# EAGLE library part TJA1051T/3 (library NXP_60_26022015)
High-speed CAN transceiver The TJA1051 is a high-speed CAN transceiver that provides an interface between a Controller Area Network (CAN) protocol controller and the physical two-wire CAN bus. The transceiver is designed for high-speed (up to 1 Mbit/s) CAN applications in the automotive industry, providing differential transmit and receive capability to (a microcontroller with) a CAN protocol controller. The TJA1051 belongs to the third generation of high-speed CAN transceivers from NXP Semiconductors, offering significant improvements over first- and second-generation devices such as the TJA1050. It offers improved ElectroMagnetic Compatibility (EMC) and ElectroStatic Discharge (ESD) performance, and also features: Ideal passive behavior to the CAN bus when the supply voltage is off TJA1051T/3 and TJA1051TK/3 can be interfaced directly to microcontrollers with supply voltages from 3 V to 5 V These features make the TJA1051 an excellent choice for all types of HS-CAN networks, in nodes that do not require a standby mode with wake-up capability via the bus. AAL Eindhoven MK
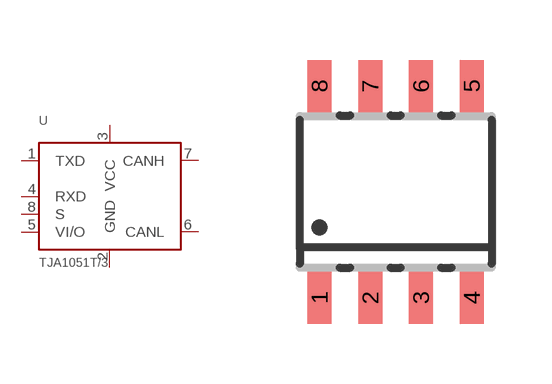
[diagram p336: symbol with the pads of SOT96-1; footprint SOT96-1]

Designator prefix U

## TJA1051T/3  [SOT96-1]
1  TXD  out
2  GND
3  VCC
4  RXD
5  VI/O  pas
6  CANL
7  CANH
8  S  pwr

## Footprint SOT96-1 (pad centres in mm)
SOT96-1 SO8: plastic small outline package; 8 leads; body width 3.9 mm JEDEC: MS-012 IEC: 076E03
smd 0.6 x 1.3: 1 -1.905,-2.65; 2 -0.635,-2.65; 3 0.635,-2.65; 4 1.905,-2.65; 5 1.905,2.65; 6 0.635,2.65; 7 -0.635,2.65; 8 -1.905,2.65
